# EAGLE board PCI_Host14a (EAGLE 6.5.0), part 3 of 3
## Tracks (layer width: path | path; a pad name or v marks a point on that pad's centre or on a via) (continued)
TRDY#  (via drill 0.2, 0.3) (continued)
  Top 0.152: 13.19,52.7 14.78,52.7 17.24,50.24 17.24,49.77 17.56,49.45 18.11,49.45 19.22,48.34 24.38,48.34 24.54,48.18 25.51,48.18 v25.75,48.42 25.67,48.34 | v58.44,77.32 57.96,76.84 57.96,73.82 58.59,73.18 58.59,71.16 58.54,71.1 58.54,67.6 v58.48,67.54
  Top 0.254: v13.11,52.7 13.11,52.78 13.19,52.7 | IC1.54 58.65,67.45 v58.48,67.54
  Top 0.305: v41.01,77.32 40.86,77.47 39.64,77.47 v39.64,77.32 | v30.19,77.32 v31.41,77.32 | v58.44,77.32 58.59,77.32
  Bottom 0.152: 9.63,51.21 10.65,52.23 12.64,52.23 v13.11,52.7 | v30.18,89.06 30.18,88.58 30.18,77.32 30.18,77.31 29.86,76.99 29.86,71.91 29.23,71.28 29.23,68.74 | v41.01,77.32 v58.44,77.32 | 29.23,68.74 | 29.23,68.74 28.91,68.42 28.91,57.78 27.16,56.04 27.16,50.48 25.75,49.07 v25.75,48.42 | v58.48,67.54 58.55,67.47 64.31,67.47 64.47,67.31 65.26,67.31 65.49,67.54 80,67.54 80.03,67.56
  Bottom 0.254: X1.J3-B12 9.63,51.21
  Bottom 0.305: 80.03,67.56 82.16,67.56 R1.4 | v31.41,77.32 v39.64,77.32 | 30.18,77.32 v30.19,77.32
TX0  (via drill 0.2, 0.3)
  Top 0.152: v48.91,47.55 49.15,48.02 IC1.3
  Top 0.305: v46.8,40.13 46.8,38 46.95,37.85 46.95,32.82 47.11,32.66 47.11,31.9 46.95,31.75 46.95,30.84 46.8,30.68 46.65,30.68 46.65,29.92 46.57,29.84 | 46.57,29.84 46.5,29.77 45.73,29.77 45.58,29.62 45.58,28.85 JP2.1 | JP2.9 55.79,28.7 55.79,25.5 55.64,25.35 46.65,25.35 46.65,29.77 46.57,29.84
  Bottom 0.152: v46.8,40.13 46.37,40.56 46.37,43.81 46.05,44.13 46.05,46.51 45.73,46.83 | 45.73,46.83 | 45.73,46.83 45.66,46.91 45.66,47.55 46.53,48.42 47.64,48.42 48.27,47.78 48.67,47.78 v48.91,47.55
  Bottom 0.305: JP2.15 63.26,28.7 62.35,28.7 62.35,29.62 62.19,29.77 61.43,29.77 61.28,29.92 60.37,29.92 60.21,29.77 58.84,29.77 58.69,29.92 57.77,29.92 57.62,29.77 57.16,29.77 57.01,29.62 56.71,29.62 56.71,28.85 56.55,28.7 55.79,28.7 JP2.9 55.64,28.7 53.2,28.7 JP2.7 | v46.8,40.13 46.65,40.13
TX1  (via drill 0.2, 0.3)
  Top 0.152: IC1.46 66.09,62.26 66.69,62.86 v66.69,63.18 66.69,63.5 66.21,63.98 66.21,65.25 67.48,66.52 67.48,70.96 67.81,71.29 v67.81,71.61
  Top 0.305: v52.59,108.56 52.74,108.41 52.74,108.26 52.9,108.1 54.27,108.1 54.27,104.6 54.42,104.45 54.42,104.29 54.57,104.14 54.73,104.14 54.88,103.99 57.01,103.99 57.01,98.04 56.86,97.89 56.86,86.98 57.32,86.52 | JP4.1 86.88,56.59 86.88,58.57 86.73,58.72 86.74,58.73 v86.74,63.76 | v57.3,72.15 57.07,72.38 57.07,73.32 57.38,73.64 57.38,81.12 57.48,81.22 57.48,86.36 57.32,86.52 | 57.32,86.52
  Bottom 0.152: 76.53,63.34 80.58,63.34 81.06,63.82 86.68,63.82 | 67.42,71.44 67.64,71.44 v67.81,71.61 | v66.69,63.18 76.37,63.18
  Bottom 0.254: 57.93,71.68 58.51,71.68 58.75,71.44 67.42,71.44
  Bottom 0.305: v52.59,108.56 52.44,108.56 52.29,108.41 51.83,108.41 51.83,108.1 51.68,107.95 39.49,107.95 39.49,109.32 39.33,109.47 38.12,109.47 J3.3 | 57.93,71.68 v57.3,72.15 | 76.37,63.18 76.53,63.34 | 86.68,63.82 v86.74,63.76
TX_USB  (via drill 0.2)
  Top 0.305: v63.26,24.43 64.02,23.67 64.02,18.49 IC3.1 | v58.38,24.43 58.54,24.59 58.54,27.48 59.6,28.55 59.6,29.16 60.82,30.38 60.82,31.14 JP2.14
  Bottom 0.305: v63.26,24.43 63.11,24.28 58.54,24.28 v58.38,24.43
V3V  (via drill 0.2, 0.3)
  Top 0.152: X1.J3-B11 X1.J3-A12 | 11.16,51.28 13.91,51.28 | v13.83,60.96 11.35,60.96 | 12.05,43.21 X1.J3-A8 | 4.14,50.22 v4.14,50.17 3.35,50.96 3.35,53.34 3.67,53.66 3.98,53.66 4.44,53.2 X1.J3-D13 X1.J3-C14 | JP6.2 13.83,15.08 15.89,13.02 17.95,13.02 18.59,13.65 v18.59,22.54
  Top 0.254: X1.J3-A12 11.16,51.28 | 13.91,51.28 v14.14,51.51 | v2.56,43.18 2.9,43.21 X1.J3-D8 | 12.05,43.21 12.12,43.14 v15.73,43.14
  Top 0.305: 11.35,60.96 X1.J3-A17 | v95.11,27.79 95.11,30.53 95.72,30.53 95.88,30.68 95.88,31.45 C31.1
  Bottom 0.152: 11.1,43.37 10.18,44.29 10.1,44.37 10.1,45.88 9.78,46.2 8.11,46.2 X1.J3-C10 | 5.06,43.21 3.98,44.29 3.98,45.88 4.3,46.2 6.08,46.2 X1.J3-C10 | X1.J3-C10 X1.J3-B11 | X1.J3-B15 X1.J3-C14 6.11,56.2 v4.14,56.2 | 13.99,51.67 13.99,60.48 | X1.J3-D17 3.83,59.94 3.83,56.52 | v4.14,50.17 2.71,50.17 2.4,49.85 2.4,43.34 v2.56,43.18 | v18.59,22.54 17,22.54 15.73,23.81
  Bottom 0.254: 5.06,43.21 X1.J3-D8 | 3.98,56.36 v4.14,56.2 3.83,56.52 | v13.83,60.96 13.83,60.64 13.99,60.48 | v14.14,51.51 13.99,51.67 | 15.73,23.81 15.73,26.87 | 15.73,26.87 v15.73,43.14 | 15.73,26.87 58.08,26.87 | 10.18,44.29
  Bottom 0.305: v95.11,27.79 80.33,27.79 80.18,27.63 73.32,27.63 73.17,27.79 64.02,27.79 63.87,27.63 63.87,27.48 61.89,27.48 61.74,27.33 61.74,27.18 58.23,27.18 58.08,27.03 58.08,26.87 | 15.73,26.87 15.71,26.87 | 11.1,43.37 11.14,43.33 X1.J3-A8
V3VIO  (via drill 0.2)
  Top 0.305: v79.26,26.26 79.26,27.33 79.87,27.33 80.03,27.48 80.03,31.14 79.87,31.29 79.87,31.9 80.03,32.05 80.03,32.21 80.18,32.21 80.33,32.36 80.33,52.78 80.79,52.78 80.94,52.93 80.94,54.15 C33.1 | v59.76,26.11 59.6,25.96 59.6,22.61 v59.76,22.45
  Bottom 0.305: v79.26,26.26 79.11,26.42 73.32,26.42 73.17,26.26 62.96,26.26 62.65,25.96 59.91,25.96 v59.76,26.11 | v59.76,22.45 59.6,22.61 24.84,22.61 JP8.2
V5V  (via drill 0.2, 0.3)
  Top 0.152: v6.13,44.21 4.22,44.21 3.67,44.77 3.35,44.77 2.08,46.04 2.08,61.59 | X1.J3-A26 12.4,79.21 12.41,79.22 13.51,79.22 13.83,78.9 14.46,78.9 | v67.8,54.61 v63.67,54.61 | v18.3,82.39 18.3,82.26 17.95,81.92 16.34,81.92 v15.86,82.39
  Top 0.254: 2.48,61.99 2.56,62.07 2.56,62.71 3.03,63.18 3.03,63.5 2.4,64.14 2.4,66.32 v2.38,66.18 | 2.48,61.99 | 2.08,61.59 2.48,61.99 | v15.73,71.28 11.16,71.28 X1.J3-A22 | 14.46,78.9 15.73,78.9 v15.81,78.98
  Top 0.305: v21.96,85.85 22.88,85.85 22.88,86.16 23.03,86.31 23.03,86.46 23.18,86.61 23.18,86.77 23.48,86.77 23.64,86.92 24.55,86.92 v24.55,87.07 | v26.99,87.07 26.99,88.14 27.14,88.29 27.9,88.29 28.21,87.99 28.21,87.83 28.36,87.68 28.51,87.68 28.51,87.53 28.67,87.38 28.82,87.38 28.82,86.16 28.97,86 30.8,86 v30.8,86.16 | v44.82,73.97 v44.82,85.85 | v52.44,59.18 52.29,59.33 52.29,63.91 52.75,64.37 v52.75,64.66 | v81.85,52.17 82.31,52.17 82.31,50.34 82.46,50.19 82.46,34.04 82.31,33.88 82.31,32.66 82.46,32.51 82.77,32.51 82.77,32.21 82.92,32.05 82.92,31.14 82.77,30.99 82.77,30.38 82.62,30.23 82.46,30.23 82.46,26.42 82.31,26.26 82.16,26.26 82.16,24.59 82.01,24.43 82.01,19.71 82.08,19.63 | 82.08,19.63 82.16,19.56 84.14,19.56 84.14,16.51 83.99,16.36 83.99,15.6 84.14,15.44 84.9,15.44 84.9,14.53 C30.1 | v11.75,19.86 11.75,21.84 JP11.2 | v15.71,19.86 v16.93,18.64 | v82.16,17.58 82.01,17.73 82.01,19.56 82.08,19.63
  Bottom 0.152: X1.J3-C1 X1.J3-D2 | 5.09,31.43 6.05,32.38 | 6.13,32.38 6.13,43.89 | 4.3,68.18 7.71,68.18 8.75,69.22 X1.J3-B21 | 3.98,68.5 3.98,71.6 4.58,72.19 | 6.29,73.82 6.13,73.66 6.13,72.27 6.07,72.21 4.6,72.21 4.58,72.19 | 6.29,73.82 | 6.29,73.82 6.76,74.3 6.76,74.88 X1.J3-C24 | 7.13,83.21 8.11,82.23 15.7,82.23 v15.86,82.39 | 8.11,82.19 X1.J3-B27 | 4.58,72.19 | 60.98,58.57 60.98,53.7 62.76,53.7 v63.67,54.61 | v67.8,54.61 67.8,53.49 68.96,52.33 81.7,52.33 v81.85,52.17 | v44.82,73.97 44.62,73.77 44.62,66.83 44.97,66.48 52.44,66.48 52.59,66.33 | 15.87,81.28 15.87,79.03 v15.81,78.98
  Bottom 0.254: X1.J3-C1 7.09,26.42 7.79,25.72 7.79,24.29 8.43,23.65 10.18,23.65 JP11.2 | X1.J3-D2 5.09,31.43 | 6.05,32.38 6.13,32.38 | 6.13,43.89 v6.13,44.21 | 4.3,68.18 3.98,68.5 3.43,67.94 2.87,67.94 2.38,67.45 v2.38,66.18 | X1.J3-B21 | v15.81,78.98 15.81,71.44 15.81,71.36 v15.73,71.28 | 7.13,83.21 X1.J3-C28 | 8.11,82.23 8.11,82.19
  Bottom 0.305: v15.86,82.39 15.87,81.28 | v18.3,82.39 18.3,83.41 18.46,83.57 20.44,83.57 20.59,83.72 20.59,85.85 v21.96,85.85 | v24.55,87.07 24.7,87.22 26.84,87.22 v26.99,87.07 | v30.8,86.16 39.03,86.16 39.18,86 44.67,86 v44.82,85.85 | v44.82,73.97 44.67,73.81 | v52.44,59.18 52.59,59.33 55.95,59.33 56.1,59.49 56.25,59.49 56.4,59.64 56.4,59.79 56.55,59.94 56.71,59.94 56.86,60.1 58.69,60.1 58.84,59.94 58.84,58.72 60.82,58.72 60.98,58.57 | v11.75,19.86 v15.71,19.86 | v16.93,18.64 23.79,18.64 23.94,18.49 31.41,18.49 31.56,18.64 32.17,18.64 32.32,18.49 39.94,18.49 40.1,18.64 54.73,18.64 56.25,17.12 60.21,17.12 60.82,17.73 61.74,17.73 61.89,17.88 78.35,17.88 78.65,17.58 v82.16,17.58 | 52.59,66.33 52.75,66.17 v52.75,64.66
V5VIO  (via drill 0.2)
  Top 0.305: v52.9,105.51 52.9,102.77 C32.1
  Bottom 0.305: v52.9,105.51 30.95,105.51 30.8,105.36 28.97,105.36 28.82,105.21 20.89,105.21 20.59,105.51 17.08,105.51 16.93,105.36 16.93,102.46 15.56,102.46 JP9.2
V5VSB  (via drill 0.2)
  Top 0.305: v9.46,24.43 9.46,2.95 v10.38,2.03 | v54.73,3.3 54.73,7.52 X3.7
  Bottom 0.152: 52.38,1.27 54.41,3.3 v54.73,3.3
  Bottom 0.305: v9.46,24.43 9.46,28.85 9.16,29.16 X1.J3-B1 | v10.38,2.03 11.14,1.27 52.38,1.27
V12M  (via drill 0.2, 0.3)
  Top 0.254: v34.46,16.66 34.46,24.3 | 39.54,25.08 39.7,25.24 42.4,25.24 42.72,25.56 v42.72,28.89 | v29.23,36.99 19.7,36.99 v18.59,38.1
  Top 0.305: v34.46,16.66 34.46,7.67 X3.3 | v22.42,89.97 22.42,89.81 19.68,89.81 19.52,89.97 19.52,93.02 C29.1 | v27.6,89.66 29.43,89.66 29.43,87.68 29.58,87.53 31.71,87.53 31.71,92.86 31.87,93.02 40.86,93.02 40.86,83.72 41.01,83.57 41.01,79.6 v41.16,79.45 | v72.56,90.27 v72.56,79.3 | v105.93,87.38 105.93,64.06 105.32,63.45 105.32,47.45 105.17,47.3 105.02,47.3 105.02,47.14 104.87,46.99 104.87,46.69 104.71,46.53 104.71,43.79 104.87,43.64 105.32,43.64 105.32,42.88 105.48,42.72 105.63,42.72 105.63,29.01 105.48,28.85 103.19,28.85 103.19,24.13 v103.04,23.98 | v61.13,12.85 v61.13,21.39 | 39.54,25.08 35.24,25.08 34.46,24.3
  Bottom 0.152: 11.1,90.14 X1.J3-A30
  Bottom 0.254: 11.1,90.14 12.08,91.12 12.87,91.12 14.3,89.69 16.21,89.69 C29.1 | v42.72,28.89 37.96,28.89 36.69,30.16 36.69,32.7 35.89,33.5 32.72,33.5 v29.23,36.99
  Bottom 0.305: v34.46,16.66 37.66,16.66 C25.+ 37.81,16.66 38.88,16.66 38.88,14.53 39.03,14.38 39.79,14.38 39.94,14.53 48.63,14.53 48.63,13 48.78,12.85 v61.13,12.85 | v22.42,89.97 24.86,89.97 25.01,89.81 25.01,89.66 v27.6,89.66 | v41.16,79.45 49.55,79.45 49.7,79.3 49.7,79.15 57.16,79.15 57.32,79.3 v72.56,79.3 | v72.56,90.27 82.46,90.27 82.62,90.42 83.22,90.42 83.38,90.58 83.99,90.58 84.14,90.42 85.66,90.42 85.82,90.27 85.82,88.9 92.52,88.9 92.67,89.05 98.77,89.05 98.92,88.9 98.92,87.22 104.87,87.22 105.02,87.38 v105.93,87.38 | v103.04,23.98 98.92,23.98 98.77,23.82 98.77,22.76 82.77,22.76 82.62,22.61 82.62,22.15 71.64,22.15 71.49,22.3 70.73,22.3 70.58,22.15 70.58,21.23 61.28,21.23 v61.13,21.39
V12P  (via drill 0.2, 0.3)
  Top 0.152: 80.33,59.49 80.33,68.48 80.79,69.09
  Top 0.254: X1.J3-A29 13.31,85.21 15.33,87.23 18.67,87.23 C28.1
  Top 0.305: v20.59,92.1 21.5,92.1 21.66,91.95 22.75,91.95 23.51,92.71 23.51,93.98 v24.3,94.77 | v28.82,96.52 28.82,96.67 27.3,96.67 27.14,96.52 27.14,96.22 27.16,96.2 v27.16,95.41 | v81.55,93.62 81.55,91.49 81.7,91.34 81.7,88.9 81.55,88.75 81.55,82.35 81.7,82.19 83.99,82.19 83.99,69.24 83.83,69.09 80.79,69.09 | 80.33,59.49 80.18,59.33 80.18,56.74 v80.33,56.59 | v71.64,56.13 71.64,53.24 71.8,53.09 71.95,53.09 71.95,39.98 71.8,39.83 71.49,39.83 v71.49,39.67 | v61.89,35.71 61.89,31.9 62.04,31.75 62.04,30.84 61.89,30.68 61.89,29.31 62.04,29.16 62.04,28.24 61.89,28.09 61.89,27.33 61.74,27.18 58.99,27.18 58.99,22.45 58.84,22.3 49.7,22.3 49.09,21.69 49.09,16.97 C24.- 49.09,16.81 v49.09,14.99 | v39.49,14.99 39.49,7.67 X3.4
  Bottom 0.305: v20.59,92.1 20.13,92.1 20.13,91.8 19.98,91.64 19.52,91.64 19.52,87.38 19.37,87.22 18.76,87.22 C28.1 | v80.33,56.59 80.18,56.44 71.8,56.44 71.64,56.29 v71.64,56.13 | v71.49,39.67 71.34,39.52 63.57,39.52 63.41,39.37 63.41,35.71 v61.89,35.71 | v24.3,94.77 26.53,94.77 v27.16,95.41 | v81.55,93.62 81.24,93.93 71.34,93.93 71.19,93.78 66.77,93.78 66.77,94.54 66.61,94.69 64.78,94.69 64.63,94.54 39.03,94.54 39.03,96.83 38.88,96.98 33.05,96.98 32.4,97.63 29.93,97.63 v28.82,96.52 | v39.49,14.99 v49.09,14.99
VCC  (via drill 0.2, 0.3)
  Top 0.152: IC1.31 60.19,54.76 59.39,55.56 55.72,55.56 | 81.7,111 82.53,111 83.04,110.49 83.04,108.74 | IC1.100 50.21,52.26 50.66,52.7 51.45,52.7 51.61,52.55 | 51.61,52.55 | v52.16,51.99 51.61,52.55
  Top 0.254: IC1.80 47.67,62.26 v48.12,62.71 | IC1.10 52.65,51.51 v52.16,51.99
  Top 0.305: JP5.2 57.16,16.66 57.01,16.81 56.25,16.81 56.25,17.12 56.1,17.27 56.1,17.73 55.95,17.88 55.95,18.64 56.1,18.8 56.1,19.56 56.25,19.71 57.16,19.71 57.16,20.78 JP10.2 | v68.14,31.6 68.14,32.97 67.98,32.97 QG1.4 | C34.1 75.45,20.32 75.45,29.62 75.61,29.77 76.06,29.77 76.06,31.45 C13.1 76.06,32.82 76.98,32.82 77.13,32.97 77.13,37.54 R2.1 77.13,37.69 77.13,47.14 78.81,47.14 78.96,47.3 78.96,48.97 IC2.16 78.96,49.12 v78.96,59.94 | v61.43,88.44 61.43,96.06 C5.1 61.43,96.22 v61.43,100.33 | R7.2 84.29,84.18 84.29,85.85 84.45,86 85.51,86 85.51,89.29 v85.11,89.69 | 81.7,111 81.55,111.15 81.55,112.06 J8.10 | J5.4 95.88,61.32 95.88,69.7 95.72,69.85 94.5,69.85 94.5,70.31 94.35,70.46 93.59,70.46 93.59,80.06 93.74,80.21 95.88,80.21 95.88,81.28 J4.4 | v46.34,100.48 46.34,103.07 JP1.2 | 55.72,55.56 v55.04,56.24 53.43,57.69 53.43,62.39 53.36,62.47 v53.36,62.71 53.59,62.71 53.67,62.63 54.86,62.63 55.15,62.91 IC1.61 55.15,73.23 C3.2 v55.42,79.85 | v49.86,88.27 v49.86,80.17 | 83.04,108.74 83.04,100.01 84.31,98.74 R3.2 R6.2 84.31,90.49 v83.68,89.85
  Bottom 0.305: JP10.2 57.16,20.78 59.6,20.78 JP10.4 59.76,20.78 73.47,20.78 73.62,20.62 73.62,20.32 C34.1 | v68.14,31.6 75.91,31.6 C13.1 77.13,31.6 77.13,30.84 77.28,30.68 78.04,30.68 78.04,30.53 78.2,30.38 83.22,30.38 83.22,31.45 83.38,31.6 84.45,31.6 C35.1 | JP1.2 46.34,103.23 44.67,103.23 44.67,103.99 44.52,104.14 41.47,104.14 41.47,103.23 41.31,103.07 40.1,103.07 C2.1 39.94,103.07 38.27,103.07 38.12,102.92 38.12,101.09 34.91,101.09 34.76,101.24 34.76,103.23 33.7,103.23 JP3.2 33.54,103.23 31.11,103.23 30.95,103.38 30.95,104.14 25.77,104.14 25.54,103.91 | 25.54,103.91 25.62,103.84 25.62,103.07 27.3,103.07 C1.1 | 25.54,103.91 25.47,103.99 20.89,103.99 20.89,103.07 20.74,102.92 19.68,102.92 C4.1 | 73.78,88.44 v61.43,88.44 61.12,88.44 60.82,88.74 54.94,88.74 54.47,88.27 v49.86,88.27 | 73.78,88.44 73.93,88.44 | J5.4 95.88,61.32 94.66,61.32 94.66,60.86 94.5,60.71 92.98,60.71 92.83,60.55 92.37,60.55 92.37,60.1 92.22,59.94 82.31,59.94 R1.1 82.16,59.94 v78.96,59.94 | J4.4 97.7,81.28 97.86,81.43 97.86,82.65 98.47,82.65 98.62,82.8 98.62,84.18 84.45,84.18 R7.2 | 74.54,88.44 80.64,88.44 80.79,88.59 81.47,88.59 82.56,89.69 | 74.54,88.44 74.08,88.44 | v46.34,100.48 46.5,100.64 55.03,100.64 55.18,100.48 55.34,100.48 55.49,100.33 v61.43,100.33 | v52.16,51.99 52.24,52.07 52.24,55.64 52.8,56.2 52.88,56.2 52.92,56.24 v55.04,56.24 | v53.36,62.71 v48.12,62.71 | v55.42,79.85 55.1,80.17 v49.86,80.17 | 82.56,89.69 | 82.56,89.69 82.72,89.85 v83.68,89.85 84.95,89.85 v85.11,89.69 | 74.54,88.44 74.39,88.29 74.23,88.29 R4.1 74.08,88.29 73.93,88.29 73.78,88.44
  pour Top (isolate 0.305): 0.01,115.57 108.6,115.57 109.23,0 1.28,0
VIO  (via drill 0.3)
  Top 0.152: X1.J3-C19 6.1,64.21 4.46,64.21 3.83,64.85 3.83,67.31 3.43,67.71 3.43,71.67 3.03,72.07 3.03,73.18 3.19,73.34 4.96,73.34 X1.J3-D23
  Top 0.254: X1.J3-A2 12.02,31.21
  Top 0.305: 12.02,31.21 v13.03,32.07
  Bottom 0.152: 14.14,42.55 14.14,50.48 14.78,51.12 14.94,51.28 14.94,51.75 14.62,52.07 14.62,65.72 14.14,66.2 10.02,66.2 | 9.94,66.2 8.51,66.2 | X1.J3-C19 8.08,66.2 8.43,66.2 | X1.J3-D23 5.09,73.5 6.13,74.53 6.13,76.04 6.29,76.2 8.09,76.2 X1.J3-B25 | X1.J3-B6 9.22,39.21 10.18,40.16 14.14,40.16 14.3,40
  Bottom 0.254: v13.03,32.07 13.03,36.51 13.83,36.51 14.14,36.83 | 14.14,36.83 | 14.14,36.83 14.3,36.99 14.3,40 14.3,42.39 14.14,42.55 | 8.51,66.2 8.43,66.2 | 10.02,66.2 9.94,66.2
XPRSNT1#  (via drill 0.2, 0.3)
  Top 0.152: 49.65,48.79 IC1.4 | 49.65,48.79 | 49.65,48.79 49.94,48.5 v49.94,47.7
  Top 0.305: v50.92,40.13 50.92,38 C7.1
  Bottom 0.152: 52.29,46.08 51.29,47.07 50.58,47.07 v49.94,47.7
  Bottom 0.305: 52.29,46.08 52.44,45.92 52.44,41.66 v50.92,40.13 | R2.8 59.3,37.69 58.08,37.69 57.93,37.54 57.93,35.86 53.36,35.86 53.2,36.02 53.2,36.78 52.74,37.24 52.14,37.24 51.98,37.39 51.98,38 51.07,38 C7.1
XPRSNT2#  (via drill 0.2, 0.3)
  Top 0.152: IC1.5 50.15,49.01 50.66,48.5 50.66,47.31 50.02,46.67 47.32,46.67 46.77,47.22 v46.46,47.22
  Top 0.305: v45.43,34.34 45.43,38.3 C8.1 | v56.86,34.34 56.86,37.54 R2.9
  Bottom 0.152: C8.1 46.37,39.37 47.48,39.37 47.64,39.53 47.64,43.66 46.54,44.76 v46.46,47.22
  Bottom 0.305: v45.43,34.34 45.58,34.49 54.42,34.49 54.57,34.34 v56.86,34.34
